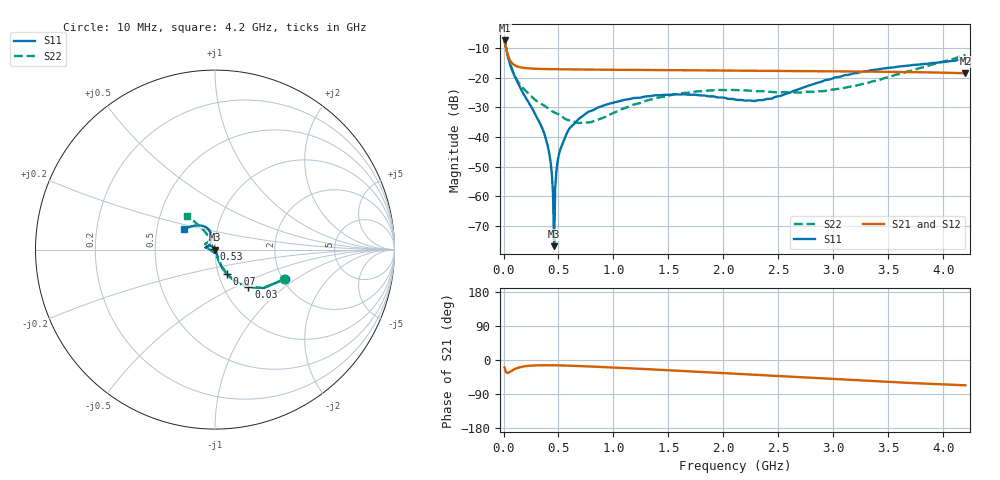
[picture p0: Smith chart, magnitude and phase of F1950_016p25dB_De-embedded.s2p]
! Integrated Device Technology
! Corporate Headquarters
! 6024 Silver Creek Valley Road
! San Jose, CA 95138  USA
! Phone:  1-408-284-8200
! Toll Free:  1-800-223-1366
! Webpage:  http://www.idt.com/
! Timing and RF Division
! 515 Groton Road, Suite 102
! Westford, MA 01886-6024
! Device:  F1950
! Description: 7-bit 0.25 dB Digital Step Attenuator
! Frequency:  150.0 -  4000.00 MHz
! Package:  4x4 mm Thin QFN Plastic Package: 24 pin
! Ports:  2 RF, 12 DC
!  Pin  1  = D0
!  Pin  2  = VDD
!  Pin  3  = Vmode
!  Pin  4  = GND
!  Pin  5  = RF1  =  Port 1
!  Pin  6  = GND
!  Pin  7  = GND
!  Pin  8  = GND
!  Pin  9  = GND
!  Pin 10  = GND
!  Pin 11  = GND
!  Pin 12  = GND
!  Pin 13  = GND
!  Pin 14  = RF2  =  Port 2
!  Pin 15  = GND
!  Pin 16  = LE
!  Pin 17  = CLK
!  Pin 18  = DATE
!  Pin 19  = D6
!  Pin 20  = D5
!  Pin 21  = D4
!  Pin 22  = D3
!  Pin 23  = D2
!  Pin 24  = D1
! State:  65
! Atten State:  16.25 dB
! Voltage:  +5.00 Volts
! Current:  Not Measured mA
! Data:  The device was measured on a the F195X evaluation board which has
!  individual transmission lines to the RF pins.  Data was collected
!  using a calibrated network analyzer.  The evaluation board was
!  de-embedded using a TRL calibration technique.
!  The reference plane is the edge of the package pin.
! Misc:  Board 2019
!  Action Tracker AT0250
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# GHz S dB R 50
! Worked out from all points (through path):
!   420 points, 10 MHz to 4.2 GHz, reference 50 ohm
!   highest |S21| = -7.32 dB at 10 MHz (marker M1); lowest = -18.4 dB at 4.2 GHz (marker M2)
!   group delay of S21, straight-line fit = 37.4 ps
!   lowest |S11| = -77.0 dB at 460 MHz (marker M3), VSWR 1.00, Z = 50 + j0.0086 ohm
!   |S11| at or under -10 dB: 23.99 MHz to end of sweep
!   |S22| runs from -35.3 to -7.5 dB; largest |S21 - S12| = 0.0002
!   S11 on the Smith chart (normalised r, x): 10 MHz: 2.06, -0.82; 30 MHz: 1.31, -0.59; 70 MHz: 1.10, -0.30; 530 MHz: 0.99, +0.01; 4.2 GHz: 0.69, +0.17
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0.01  -7.47 -22.6  -7.32 -20.0  -7.32 -20.0  -7.52 -23.1
0.03  -11.10 -48.1  -10.95 -33.8  -10.94 -33.8  -11.06 -48.3
0.07  -16.55 -64.1  -14.67 -29.2  -14.67 -29.2  -16.30 -63.7
0.16  -23.94 -70.1  -16.46 -18.4  -16.46 -18.4  -22.71 -71.1
0.37  -38.76 -61.8  -16.99 -13.8  -16.99 -13.8  -29.38 -78.5
0.42  -46.43 -64.0  -17.03 -13.8  -17.03 -13.8  -30.70 -80.5
0.43  -49.10 -65.0  -17.04 -13.8  -17.04 -13.9  -30.95 -81.5
0.44  -52.71 -65.2  -17.05 -13.9  -17.04 -13.9  -31.22 -82.9
0.46  -76.97 142.7  -17.06 -14.0  -17.05 -14.0  -31.65 -85.7
0.48  -51.96 122.0  -17.07 -14.1  -17.07 -14.1  -31.97 -88.1
0.49  -48.71 123.2  -17.07 -14.1  -17.07 -14.1  -32.12 -89.1
0.5  -46.61 125.3  -17.08 -14.2  -17.08 -14.2  -32.29 -89.8
0.53  -42.89 128.9  -17.09 -14.4  -17.09 -14.4  -33.00 -91.7
0.6  -37.12 130.8  -17.12 -15.0  -17.12 -15.0  -34.36 -104.7
0.71  -33.15 134.9  -17.16 -16.2  -17.15 -16.2  -35.18 -124.7
0.99  -28.45 146.1  -17.25 -19.8  -17.24 -19.8  -32.04 -171.1
1.41  -25.87 163.0  -17.35 -25.7  -17.35 -25.7  -26.65 166.3
2.11  -27.35 158.5  -17.52 -36.3  -17.51 -36.3  -24.16 148.3
2.43  -27.06 126.0  -17.59 -41.1  -17.59 -41.2  -24.72 138.5
2.81  -22.23 104.8  -17.69 -47.2  -17.69 -47.2  -24.73 123.5
3.51  -16.55 117.4  -17.94 -57.9  -17.93 -57.9  -19.71 118.3
4.2  -13.53 146.3  -18.41 -66.7  -18.41 -66.8  -12.22 129.4
